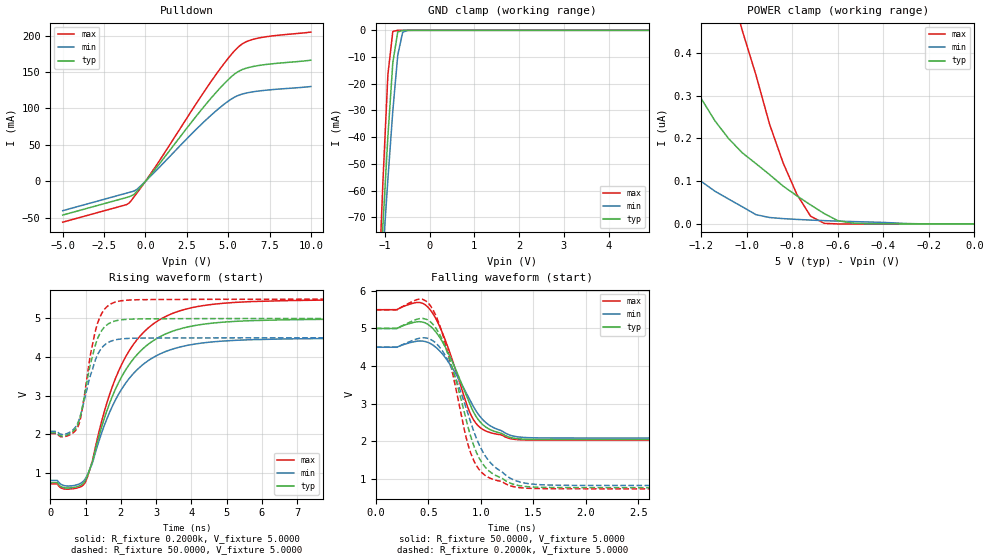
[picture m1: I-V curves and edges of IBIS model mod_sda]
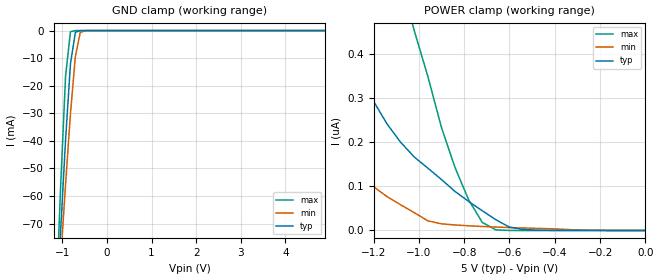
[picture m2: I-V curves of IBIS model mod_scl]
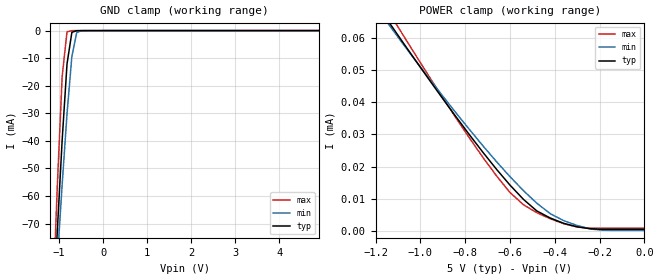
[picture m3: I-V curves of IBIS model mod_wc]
| IBIS (I/O, Buffer, Information, Specification) Model, officially
| electronic behavioral standard for Buffer structures of digital pins.
[IBIS ver]  4.0
[File name] m24m02e_5d0_dfn8.ibs
[File Rev]  1.0
[Date]   10 May 2023
[Source]   CAD & Design Services (Catania) - STMicroelectronics
[Notes]
   (Note1)  This IBIS model includes the DFN8 package parasitic data
   (Note2)  This IBIS model has some Notes about the non-monotonicity
   of the I-V curves, but they are not indicative of problems
   inside the model;
[Disclaimer]
   Customers are solely responsible for all aspects of their
   own product designs or applications using this IBIS Model.
   STMicroelectronics assumes no liability for Custmer Designs
   and applications associated to this IBIS Model.
   In the use of this IBIS Model Customer shall not modify,
   disassemble, alter this Model in whole or in part.
   If Customers do not accept these terms, the IBIS Model
   may not be used. For any problems or modifications please
   contact STMicroelectronics (www.st.com).
[Copyright] (c) 2023 STMicroelectronics
|   Component M24m02e
[Component] M24m02e
[Manufacturer] STMicroelectronics
[Package]
| variable   typ   min   max
R_pkg   0.0   0.0   0.0
L_pkg   0.0H   0.0H   0.0H
C_pkg   0.0F   0.0F   0.0F
[Pin]  signal_name   model_name   R_pin   L_pin   C_pin
1   DU   NC   0.0   0.0   0.0
2   E2   mod_en   0.0   0.0   0.0
3   E3   mod_en   0.0   0.0   0.0
4   VSS   GND   0.0   0.0   0.0
5   SDA   mod_sda   0.0   0.0   0.0
6   SCL   mod_scl   0.0   0.0   0.0
7   WC   mod_wc   0.0   0.0   0.0
8   VCC   POWER   0.0   0.0   0.0
[Package Model]  182694_DFN8   | also called 182694_MLP_2x3
[Define Package Model]  182694_DFN8
[Manufacturer]  STMicroelectronics
[OEM]  STMicroelectronics
[Description]  8 pin DFN8 2x3
[Number Of Pins]  8
[Pin Numbers]
|Pin Num   Terminal Name
1   | net1
2   | net2
3   | net3
4   | net4_GND
5   | net5
6   | net6
7   | net7
8   | net8_VDD
[Model Data]
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[End Model Data]
[End Package Model]
| Models and submodels in the file (4): mod_sda (I/O_open_drain), mod_scl (Input), mod_wc (Input), mod_en (Input)
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|   Model mod_sda
[Model]   mod_sda
Model_type I/O_open_drain
Polarity   Inverting
Enable   Active-High
Vinl   =   1.500V
Vinh   =   3.500V
Vmeas  =   2.500V
Cref   =   30pF
Rref   =   500
Vref   =   5.000V
C_comp   4.636pF   4.427pF   4.856pF
[Temperature Range]  25.0000   85.0000   -40.0000
[Voltage Range]   5.0000V   4.5000V   5.5000V
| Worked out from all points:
|   slope of the pulldown table from 0 to 0.75 V, typ, clamps not added: 35.3 ohm
|   GND clamp passes 1 mA (typ) near -0.71 V on its own axis
|   rising waveform, R_fixture 0.2000k, V_fixture 5.0000: 20-80 % time 1.26ns typ, 1.27ns min, 1.26ns max; typ from 0.75 V to 4.99 V
|   rising waveform, R_fixture 50.0000, V_fixture 5.0000: 20-80 % time 420ps typ, 440ps min, 398ps max; typ from 2.04 V to 5 V
|   falling waveform, R_fixture 50.0000, V_fixture 5.0000: 20-80 % time 282ps typ, 308ps min, 257ps max; typ from 5 V to 2.04 V
|   falling waveform, R_fixture 0.2000k, V_fixture 5.0000: 20-80 % time 268ps typ, 308ps min, 238ps max; typ from 5 V to 0.751 V
[Pulldown]
|Voltage   I(typ)   I(min)   I(max)
-5V       -46.32mA   -40.32mA   -56.11mA
-1V       -21.32mA   -15.32mA   -30.1mA
-680mV    -17.9mA    -13.22mA   -21.04mA
-360mV    -9.73mA    -7.876mA   -11.37mA
760mV     21.55mA    17.37mA    25.35mA
2.84V     82.84mA    66.22mA    98.7mA
4.12V     118.2mA    93.82mA    142mA
5.08V     141.3mA    111.3mA    171.1mA
5.72V     152.1mA    118.8mA    186.5mA
6.2V      156.1mA    121.7mA    192.7mA
6.84V     159mA      124mA      196.7mA
10V       166.3mA    130.2mA    204.9mA
[GND_clamp]
|Voltage   I(typ)   I(min)   I(max)
-5V       -1.422A    -1.176A    -1.866A
-1.15V    -107.2mA   -111.7mA   -101.9mA
-1.04V    -72.5mA    -83.27mA   -56.29mA
-930mV    -39.66mA   -55.77mA   -16.56mA
-820mV    -12.07mA   -30.13mA   -402.8uA
-710mV    -609.6uA   -9.335mA   -4.14uA
-600mV    -10.22uA   -717.4uA   -32.48nA
-490mV    -151.4nA   -22.68uA   -140.4pA
4.9V      24.41pA    1.481nA    23.56pA
[POWER_clamp]
|Voltage   I(typ)   I(min)   I(max)
-4.98V    22.67uA    13.45uA    39.59uA
-1.8V     927nA      454.3nA    3.005uA
-1.62V    682nA      304.3nA    2.197uA
-1.38V    447.3nA    168.6nA    1.383uA
-1.14V    240.9nA    76.49nA    697.7nA
-1.02V    166.3nA    40.21nA    452.1nA
-900mV    115.3nA    15.06nA    232.9nA
-840mV    88.27nA    12.47nA    142nA
-780mV    65.71nA    10.63nA    69.1nA
-720mV    44.6nA     9.087nA    18.24nA
-540mV    2.332nA    5.661nA    40.22pA
0V        24.99pA    35.71pA    26.88pA
[Ramp]
| variable   typ   min   max
dV/dt_r  1.7772/0.4957n   1.4534/0.5134n   2.0879/0.4753n
dV/dt_f  1.7776/0.3030n   1.4537/0.3605n   2.0883/0.2757n
R_load = 50.0000
[Rising Waveform]
R_fixture= 0.2000k
V_fixture= 5.0000
V_fixture_min= 4.5000
V_fixture_max= 5.5000
|time   V(typ)   V(min)   V(max)
0s        749.7mV    806.9mV    717.9mV
510ps     610.3mV    661.5mV    581.2mV
990ps     799.4mV    844mV      752.9mV
1.19ns    1.276V     1.246V     1.299V
1.61ns    2.623V     2.414V     2.828V
2.01ns    3.467V     3.15V      3.782V
2.55ns    4.147V     3.746V     4.546V
3.23ns    4.579V     4.127V     5.03V
5.23ns    4.921V     4.431V     5.412V
10ns      4.988V     4.488V     5.488V
[Rising Waveform]
R_fixture= 50.0000
V_fixture= 5.0000
V_fixture_min= 4.5000
V_fixture_max= 5.5000
|time   V(typ)   V(min)   V(max)
0s        2.037V     2.077V     2.019V
440ps     1.971V     2.009V     1.948V
780ps     2.257V     2.292V     2.19V
900ps     2.66V      2.634V     2.61V
1.12ns    3.742V     3.468V     3.967V
1.3ns     4.371V     3.974V     4.747V
1.5ns     4.737V     4.277V     5.188V
1.78ns    4.916V     4.428V     5.401V
2.66ns    4.987V     4.49V      5.484V
10ns      4.999V     4.499V     5.499V
[Falling Waveform]
R_fixture= 50.0000
V_fixture= 5.0000
V_fixture_min= 4.5000
V_fixture_max= 5.5000
|time   V(typ)   V(min)   V(max)
0s        5V         4.5V       5.5V
400ps     5.18V      4.664V     5.695V
490ps     5.12V      4.635V     5.585V
570ps     4.913V     4.503V     5.27V
670ps     4.461V     4.193V     4.63V
870ps     3.156V     3.232V     2.945V
930ps     2.778V     2.917V     2.57V
1.05ns    2.368V     2.487V     2.265V
1.31ns    2.078V     2.133V     2.05V
10ns      2.037V     2.077V     2.019V
[Falling Waveform]
R_fixture= 0.2000k
V_fixture= 5.0000
V_fixture_min= 4.5000
V_fixture_max= 5.5000
|time   V(typ)   V(min)   V(max)
0s        5V         4.5V       5.5V
420ps     5.265V     4.743V     5.784V
520ps     5.177V     4.711V     5.606V
600ps     4.882V     4.528V     5.148V
680ps     4.369V     4.185V     4.409V
860ps     2.571V     2.88V      2.096V
940ps     1.823V     2.206V     1.439V
1.08ns    1.199V     1.461V     1.021V
1.34ns    827.1mV    936.7mV    770mV
10ns      750.6mV    808.2mV    718.6mV
|   Model mod_scl
[Model]   mod_scl
Model_type Input
Vinl   =   1.500V
Vinh   =   3.500V
C_comp   3.062pF   2.954pF   3.207pF
[Temperature Range]  25.0000   85.0000   -40.0000
[Voltage Range]   5.0000V   4.5000V   5.5000V
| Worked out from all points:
|   GND clamp passes 1 mA (typ) near -0.71 V on its own axis
[GND_clamp]
|Voltage   I(typ)   I(min)   I(max)
-5V       -1.422A    -1.176A    -1.866A
-1.15V    -107.2mA   -111.7mA   -101.9mA
-1.04V    -72.5mA    -83.27mA   -56.29mA
-930mV    -39.66mA   -55.77mA   -16.56mA
-820mV    -12.07mA   -30.13mA   -402.8uA
-710mV    -609.6uA   -9.335mA   -4.14uA
-600mV    -10.22uA   -717.4uA   -32.48nA
-490mV    -151.4nA   -22.68uA   -140.4pA
4.9V      24.41pA    1.481nA    23.56pA
[POWER_clamp]
|Voltage   I(typ)   I(min)   I(max)
-4.98V    22.67uA    13.45uA    39.59uA
-1.8V     927nA      454.3nA    3.005uA
-1.62V    682nA      304.3nA    2.197uA
-1.38V    447.3nA    168.6nA    1.383uA
-1.14V    240.9nA    76.49nA    697.7nA
-1.02V    166.3nA    40.21nA    452.1nA
-900mV    115.3nA    15.06nA    232.9nA
-840mV    88.27nA    12.47nA    142nA
-780mV    65.71nA    10.63nA    69.1nA
-720mV    44.6nA     9.087nA    18.24nA
-540mV    2.332nA    5.661nA    40.22pA
0V        24.99pA    35.71pA    26.88pA
|   Model mod_wc
[Model]   mod_wc
Model_type Input
Vinl   =   1.500V
Vinh   =   3.500V
C_comp   3.062pF   2.954pF   3.207pF
[Temperature Range]   25.0000   85.0000   -40.0000
[Voltage Range]   5.0000V   4.5000V   5.5000V
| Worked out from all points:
|   GND clamp passes 1 mA (typ) near -0.71 V on its own axis
[GND_clamp]
|Voltage   I(typ)   I(min)   I(max)
-5V       -1.422A    -1.176A    -1.866A
-1.15V    -107.2mA   -111.7mA   -101.9mA
-1.04V    -72.5mA    -83.27mA   -56.29mA
-930mV    -39.66mA   -55.77mA   -16.57mA
-820mV    -12.07mA   -30.13mA   -418.3uA
-710mV    -620.9uA   -9.339mA   -20.79uA
-600mV    -22.36uA   -725.8uA   -12.57uA
-490mV    -9.416uA   -31.56uA   -9.594uA
4.9V      4.491uA    3.191uA    11.44uA
[POWER_clamp]
|Voltage   I(typ)   I(min)   I(max)
-4.98V    513.8uA    484.9uA    553uA
-1.14V    64.86uA    64.06uA    67.95uA
-1.08V    58.82uA    58.4uA     61.2uA
-900mV    41.11uA    41.92uA    41.41uA
-720mV    24.37uA    26.4uA     22.77uA
-600mV    14.24uA    16.87uA    11.94uA
-540mV    9.813uA    12.52uA    8.144uA
-480mV    6.196uA    8.6uA      5.646uA
-420mV    4.001uA    5.357uA    3.773uA
-300mV    1.259uA    1.679uA    1.234uA
-180mV    449.5nA    204.6nA    834.4nA
0V        449.4nA    139.2nA    834.4nA
